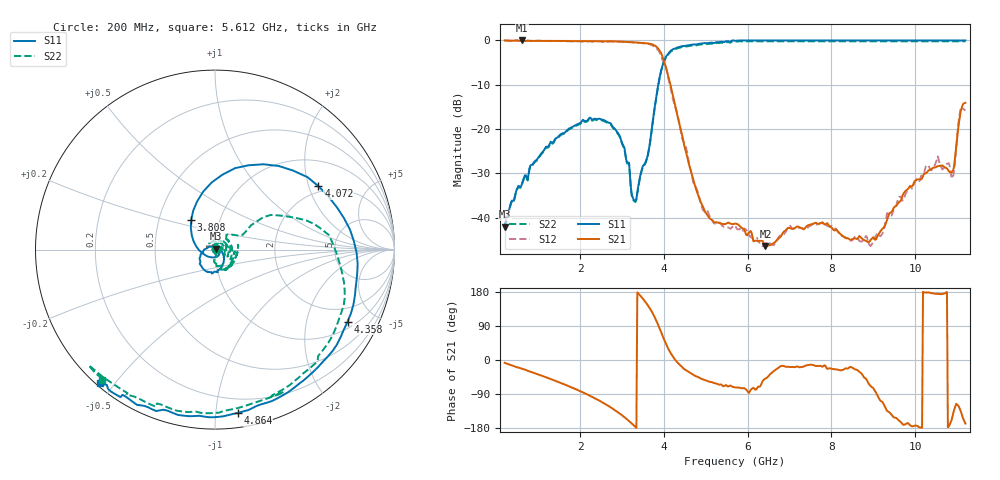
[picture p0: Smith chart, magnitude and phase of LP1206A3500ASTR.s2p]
!	AVX	THIN	FILM	OPERATION
!	LP1206	High	Performance	Low	Pass	Filters
!	P/N	LP1206A3500ASTR	18	October	2017
!Instrument:	"HEWLETT PACKARD,8720ES,US39172150,7.62 "
#	MHz	S	dB	R	50
!	Frq	S11(dB)	S11(deg)	S21(dB)	S21(deg)	S12(dB)	S12(deg)	S22(dB)	S22(deg)
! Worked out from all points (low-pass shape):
!   501 points, 200 MHz to 11.2 GHz, reference 50 ohm
!   highest |S21| = 0.00 dB at 618 MHz (marker M1); lowest = -46.4 dB at 6.426 GHz (marker M2)
!   |S21| within 3 dB of the highest: start of sweep to 3.943 GHz
!   lowest |S11| = -42.0 dB at 200 MHz (marker M3), VSWR 1.02, Z = 50.6 + j0.501 ohm
!   |S11| at or under -10 dB: start of sweep to 3.867 GHz
!   |S22| runs from -42.2 to -0.2 dB; largest |S21 - S12| = 0.065
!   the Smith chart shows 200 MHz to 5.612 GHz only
!   S11 on the Smith chart (normalised r, x): 200 MHz: 1.01, +0.01; 3.808 GHz: 0.73, +0.25; 4.072 GHz: 1.79, +2.32; 4.358 GHz: 1.28, -3.50; 4.864 GHz: 0.10, -1.14; 5.612 GHz: 0.01, -0.46
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200  -42.05 38.8  0.00 -7.5  -0.05 -7.3  -42.25 36.2
618  -32.22 -3.8  0.00 -23.3  -0.04 -23.2  -32.42 44.3
2048  -18.18 -83.5  -0.15 -84.3  -0.26 -84.5  -18.38 -43.4
2906  -20.90 -155.3  -0.23 -137.9  -0.31 -137.3  -21.10 -92.5
3302  -36.11 68.6  -0.43 -174.5  -0.49 -174.4  -36.31 -37.3
3588  -26.83 -105.7  -0.64 149.2  -0.64 148.4  -27.03 91.9
3808  -13.50 128.8  -1.30 107.0  -1.68 106.0  -13.70 31.1
3874  -9.63 101.5  -1.95 90.4  -2.29 89.4  -9.83 34.0
4072  -3.40 31.5  -6.83 38.0  -6.90 38.6  -3.60 2.2
4358  -1.51 -28.5  -18.29 -10.2  -18.10 -9.2  -1.71 -42.7
4864  -0.74 -82.1  -36.09 -47.9  -36.08 -51.0  -0.94 -85.6
5612  -0.16 -130.6  -41.40 -68.7  -42.32 -69.3  -0.36 -130.8
5700  -0.08 -136.4  -41.34 -72.3  -41.74 -72.6  -0.28 -139.9
6426  0.00 -174.4  -46.38 -48.9  -46.21 -41.7  -0.20 -168.9
7548  0.00 130.6  -41.43 -12.8  -41.56 -12.8  -0.20 138.9
8208  0.00 100.0  -43.63 -26.9  -43.83 -23.8  -0.20 110.8
8934  0.00 67.2  -45.08 -68.3  -46.41 -69.4  -0.20 81.6
9374  0.00 49.2  -39.30 -137.2  -39.07 -140.1  -0.20 70.3
10276  0.00 9.0  -29.84 177.9  -28.13 -176.4  -0.20 25.0
10870  0.00 -18.0  -29.86 -158.5  -31.23 -171.7  -0.20 -10.0
11068  0.00 -26.4  -17.20 -129.3  -16.40 -133.5  -0.20 -13.2
11200  0.00 -29.6  -14.07 -167.7  -15.82 -166.4  -0.20 -2.3
